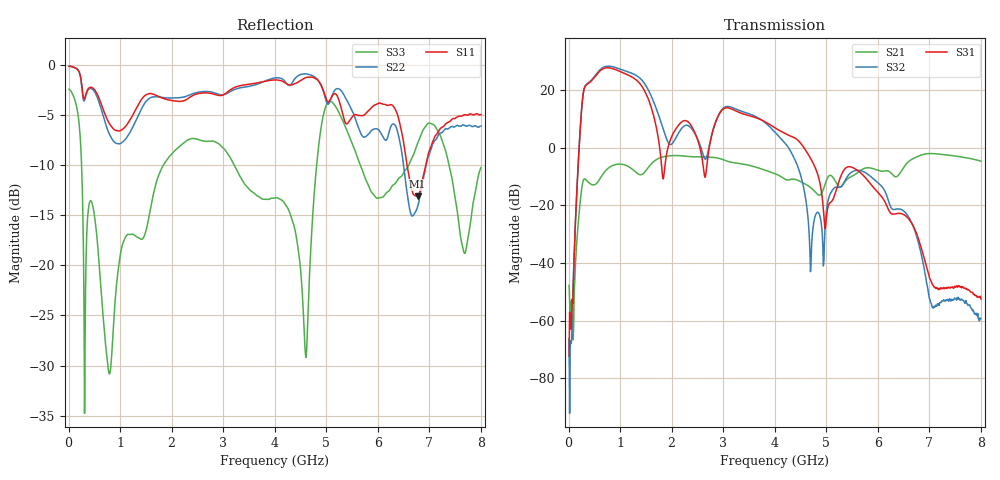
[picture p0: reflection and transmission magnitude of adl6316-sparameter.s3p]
!Agilent Technologies,N5222A,MY51421716,A.10.20.01
!Agilent N5222A: A.10.20.01
!Date: Wednesday, February 20, 2019 14:32:32
!Correction: S11(Full 3 Port(1,2,3))
!S12(Full 3 Port(1,2,3))
!S13(Full 3 Port(1,2,3))
!S21(Full 3 Port(1,2,3))
!S22(Full 3 Port(1,2,3))
!S23(Full 3 Port(1,2,3))
!S31(Full 3 Port(1,2,3))
!S32(Full 3 Port(1,2,3))
!S33(Full 3 Port(1,2,3))
!S3P File: Measurements: <S11,S12,S13>,
!<S21,S22,S23>,
!<S31,S32,S33>:
# Hz S  dB  R 50
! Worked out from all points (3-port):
!   801 points, 10 MHz to 8 GHz, reference 50 ohm
!   strongest paths, dB at 10 MHz, 2.007 GHz, 4.005 GHz, 6.003 GHz, 8 GHz:
!     S31: -72.3, 4.2, 6.9, -15.5, -52.4
!     S32: -66.2, 1.4, 5.4, -12.1, -59.2
!     S21: -47.7, -2.7, -9.0, -7.8, -4.6
!   lowest |S11| = -13.1 dB at 6.772 GHz (marker M1), VSWR 1.57, Z = 32.7 + j5.86 ohm
!   |S11| at or under -10 dB: 6.567 GHz to 6.932 GHz (365.1 MHz wide, 5.41 % of centre)
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1e7  -0.16 178.6  -47.72 -16.6  -71.55 51.3
     -47.74 -11.8  -0.14 178.5  -73.74 -44.8
     -72.26 130.7  -66.24 -132.8  -2.42 174.0
5.593125e8  -2.96 109.8  -11.99 81.3  -67.92 128.5
            -12.03 81.7  -3.27 109.0  -67.42 -51.1
            25.73 -17.0  26.07 161.0  -17.72 -37.0
6.8915e8  -4.69 92.2  -8.57 74.0  -63.65 52.6
          -8.56 74.2  -5.42 92.1  -62.47 -132.7
          27.58 -95.0  28.05 82.6  -26.30 -57.8
8.389625e8  -6.21 77.6  -6.30 52.7  -61.24 -35.0
            -6.29 52.8  -7.36 81.3  -60.23 137.7
            27.55 -176.9  28.18 0.6  -28.73 -0.0
1.018738e9  -6.53 56.6  -5.69 28.7  -60.50 -121.9
            -5.69 28.7  -7.81 65.5  -59.36 52.1
            26.33 97.7  27.20 -84.2  -18.49 -22.9
1.218488e9  -5.26 23.2  -7.19 9.9  -59.99 141.8
            -7.20 9.9  -6.47 35.4  -58.64 -37.4
            24.66 8.2  25.92 -171.6  -16.90 -62.0
1.558062e9  -2.87 -47.5  -6.56 29.2  -65.88 -12.8
            -6.56 29.2  -3.38 -35.9  -63.86 169.3
            16.40 -155.7  19.70 32.5  -15.19 -67.3
4.005e9  -1.50 -166.0  -8.98 -99.6  -70.40 -41.2
         -8.99 -99.6  -1.30 -170.4  -71.46 137.2
         6.93 -88.5  5.40 89.4  -13.28 -143.9
6.771538e9  -13.12 157.3  -3.04 -94.0  -64.00 164.3
            -3.04 -93.9  -14.16 157.4  -65.63 147.0
            -30.74 -18.0  -31.81 -19.2  -7.83 -166.1
8e9  -4.96 118.1  -4.64 -174.3  -62.82 165.7
     -4.64 -174.3  -6.11 93.6  -63.35 160.9
     -52.45 141.3  -59.23 137.6  -10.24 -117.3
